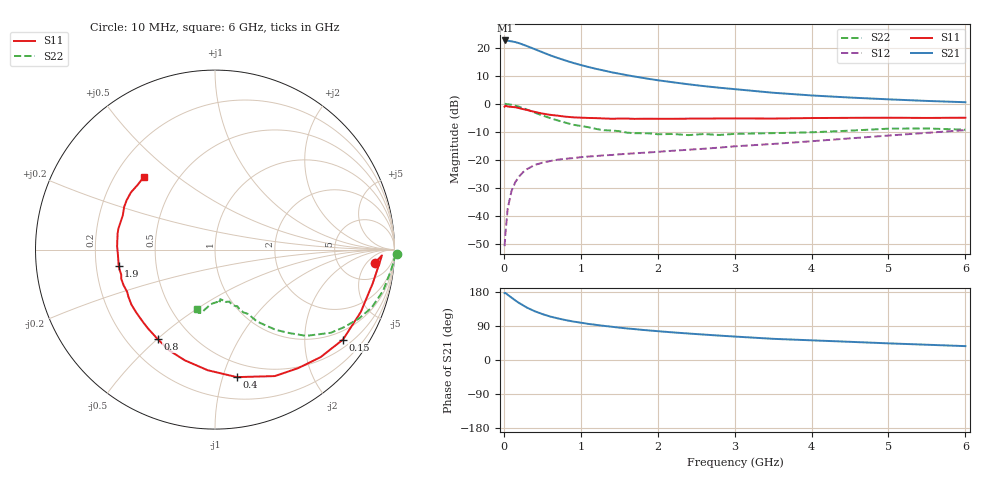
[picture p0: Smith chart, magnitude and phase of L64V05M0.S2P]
!  INFINEON TECHNOLOGIES Small Signal Semiconductors
! BFR380L3 , Si-NPN RF-Transistor in TSLP-3-1
!  Vce=4 V,  Ic=5 mA
! Common Emitter S-Parameters:  07. March 2005
#  GHz  S  MA  R  50
! f  S11  S21  S12  S22
! GHz  Mag  Ang  Mag  Ang  Mag  Ang  Mag  Ang
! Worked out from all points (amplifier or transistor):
!   36 points, 10 MHz to 6 GHz, reference 50 ohm
!   highest |S21| = 22.6 dB at 20 MHz (marker M1)
!   |S21| within 3 dB of that: start of sweep to 392.1 MHz
!   unconditionally stable (mu >= 1): 2.608 GHz to 4.647 GHz
!   at 250 MHz: K = 0.16, MSG = 22.8 dB, |S12| = -24.4 dB
!   at 1.4 GHz: K = 0.74, MSG = 14.8 dB, |S12| = -18.2 dB
!   at 6 GHz: K = 0.93, MSG = 5.0 dB, |S12| = -9.4 dB
!   S11 on the Smith chart (normalised r, x): 10 MHz: 11, -8; 150 MHz: 0.72, -3.01; 400 MHz: 0.38, -1.11; 800 MHz: 0.33, -0.50; 1.9 GHz: 0.30, -0.08; 6 GHz: 0.32, +0.38
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0.01  0.8919 -4.8  13.53 176.6  0.0029 79.5  1.012 -1.4
0.02  0.9308 -2.0  13.54 177.1  0.0047 88.5  1.001 -2.9
0.05  0.8989 -12.0  13.39 172.1  0.0136 85.2  0.9866 -7.0
0.1  0.8835 -23.2  13.03 164.6  0.0281 79.0  0.9643 -13.8
0.15  0.8716 -35.1  12.66 157.1  0.0404 72.0  0.9309 -20.3
0.2  0.8397 -45.5  12.07 150.2  0.051 68.1  0.8891 -25.6
0.25  0.8069 -54.9  11.42 144.3  0.0605 62.3  0.8382 -31.1
0.3  0.7795 -64.7  10.75 138.3  0.0684 59.0  0.7943 -35.7
0.4  0.7208 -80.3  9.492 128.8  0.0813 52.7  0.6995 -43.4
0.5  0.6732 -93.5  8.358 121.3  0.0893 48.4  0.6229 -48.3
0.6  0.6393 -105.3  7.381 114.8  0.0955 45.5  0.5602 -52.9
0.8  0.592 -122.7  5.951 105.4  0.105 42.2  0.4637 -59.7
0.9  0.5765 -130.4  5.39 101.6  0.1079 41.5  0.4249 -61.6
1.1  0.5615 -141.4  4.552 95.2  0.1152 41.4  0.3835 -65.7
1.5  0.5466 -158.6  3.456 85.4  0.126 42.9  0.3262 -72.0
1.9  0.5442 -170.6  2.773 77.8  0.1365 45.6  0.2977 -78.3
2.2  0.5418 -177.6  2.428 72.8  0.1461 47.9  0.2904 -80.0
2.8  0.5499 170.5  1.945 64.4  0.166 52.5  0.2793 -87.3
3.5  0.5479 159.7  1.582 55.9  0.1932 55.5  0.3009 -92.8
4.5  0.564 150.7  1.298 48.0  0.2428 60.0  0.3333 -98.9
5.5  0.5619 140.3  1.13 40.3  0.3047 60.8  0.3644 -104.5
6  0.5671 134.2  1.071 36.6  0.3407 60.0  0.3467 -107.2
